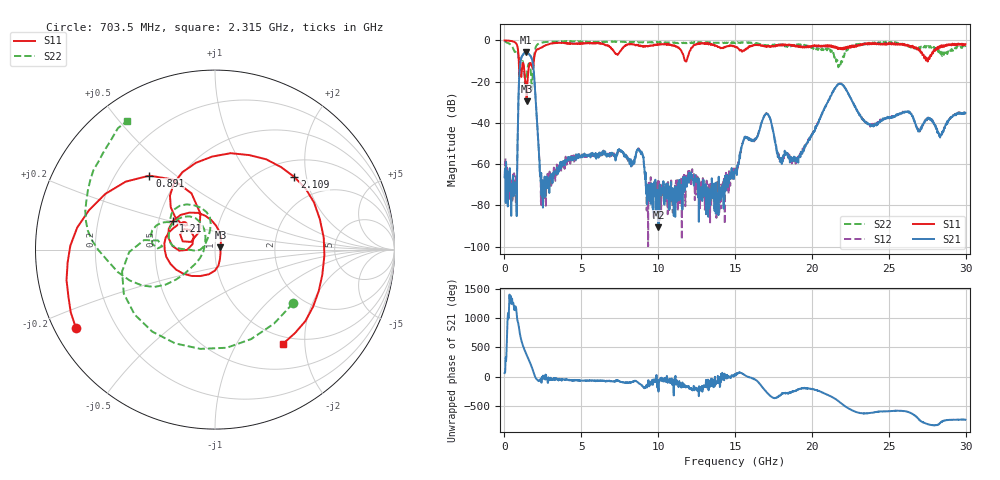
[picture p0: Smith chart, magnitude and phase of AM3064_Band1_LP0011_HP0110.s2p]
# Hz S DB R 50.0
!freq dBS11 angS11 dBS21 angS21 dBS12 angS12 dBS22 angS22
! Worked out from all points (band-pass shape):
!   1600 points, 10 MHz to 29.98 GHz, reference 50 ohm
!   highest |S21| = -5.69 dB at 1.397 GHz (marker M1); lowest = -90.6 dB at 10.02 GHz (marker M2)
!   |S21| within 3 dB of the highest: 1.089 GHz to 1.767 GHz (678.3 MHz wide, 47.5 % of centre)
!   lowest |S11| = -29.6 dB at 1.435 GHz (marker M3), VSWR 1.07, Z = 53.1 + j1.41 ohm
!   |S11| at or under -10 dB: 931.4 MHz to 1.914 GHz (982.2 MHz wide, 69 % of centre); 11.76 GHz to 11.84 GHz (85.55 MHz wide, 0.725 % of centre); 27.52065 GHz to 27.5489 GHz (28.25 MHz wide, 0.103 % of centre)
!   |S22| runs from -24.0 to -0.3 dB; largest |S21 - S12| = 0.0063
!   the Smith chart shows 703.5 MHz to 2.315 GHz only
!   S11 on the Smith chart (normalised r, x): 703.5 MHz: 0.06, -0.26; 891 MHz: 0.34, +0.41; 1.21 GHz: 0.59, +0.21; 2.109 GHz: 1.35, +1.70; 2.315 GHz: 0.88, -1.59
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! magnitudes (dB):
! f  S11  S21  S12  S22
! 10 MHz  0.0  -66.4  -60.4  -0.3
! 703.5 MHz  -1.0  -68.9  -68.5  -5.5
! 891 MHz  -5.2  -35.5  -35.4  -6.4
! 1.21 GHz  -11.0  -6.9  -6.8  -10.5
! 1.397 GHz  -22.6  -5.7  -5.7  -21.7
! 1.435 GHz  -29.6  -5.7  -5.7  -18.5
! 1.828 GHz  -13.5  -10.4  -10.3  -17.7
! 2.109 GHz  -4.5  -38.0  -38.1  -2.3
! 2.315 GHz  -3.8  -65.5  -66.0  -1.2
! 2.559 GHz  -2.7  -71.2  -73.6  -0.8
! 5.015 GHz  -1.4  -55.9  -56.0  -0.8
! 8.763 GHz  -2.8  -53.1  -53.1  -1.0
! 9.344 GHz  -2.9  -72.6  -99.8  -0.9
! 10 GHz  -2.0  -73.1  -75.1  -0.9
! 10.02 GHz  -1.9  -90.6  -70.1  -0.9
! 15 GHz  -3.0  -64.1  -62.8  -1.4
! 17.01 GHz  -3.2  -35.5  -35.5  -2.5
! 17.95 GHz  -2.3  -59.0  -57.8  -2.0
! 19.99 GHz  -3.1  -45.9  -46.2  -3.4
! 21.81 GHz  -4.1  -21.1  -21.1  -12.7
! 25 GHz  -1.4  -37.2  -37.2  -1.0
! 29.98 GHz  -1.8  -35.2  -35.2  -3.2
